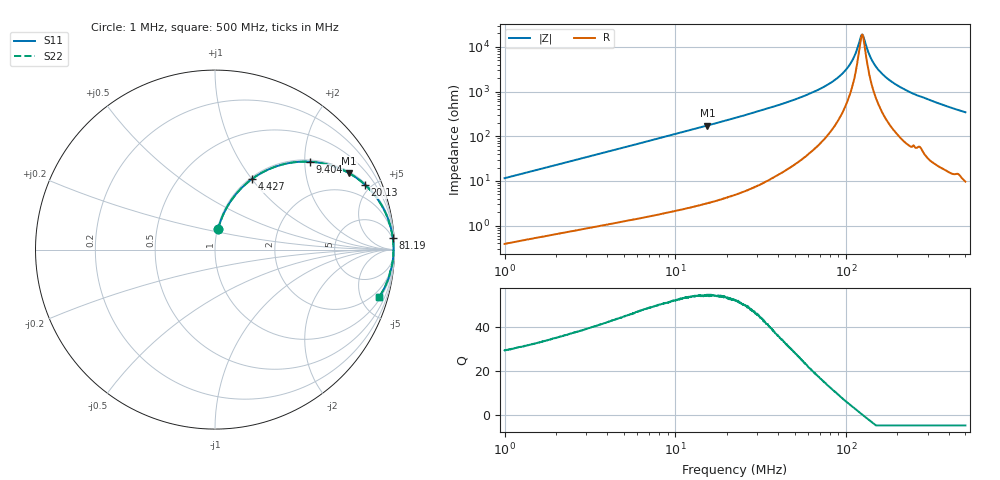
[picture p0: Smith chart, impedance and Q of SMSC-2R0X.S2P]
!s-Parameter Generated by FASTRON Sdn. Bhd.
!FASTRON P/N : SMSC-2R0X
!Keysight Technologies,E4991B,MY54100416,A.01.15
!Date: Mon Mar 16 10:09:13 2026
!Version  : Rev00 Mon Mar 16 10:09:13 2026
!Data & Calibration Information:
!PortZ  Port1:50+j0  Port2:50+j0
!When reading, reference impedance value at option line is always used.
! Remarks : This data is being provided solely for informational purposes.
!Freq	S11	S21	S12	S22
# Hz S dB R 50
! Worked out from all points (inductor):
!   1601 points, 1 MHz to 500 MHz, reference 50 ohm
!   read as one part in series: L = 1.83 uH near 1.032 MHz
!   highest Q = 54.8 at 15.4 MHz (marker M1), where L = 1.8 uH
!   self-resonance near 124 MHz
!   S11 on the Smith chart (normalised r, x): 1 MHz: 1.01, +0.23; 4.427 MHz: 1.02, +1.00; 9.404 MHz: 1.04, +2.11; 20.13 MHz: 1.09, +4.59; 81.19 MHz: 4, +31; 500 MHz: 1.19, -6.89
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1000000  -18.84 81.5  -0.09 -6.6  -0.09 -6.6  -18.84 81.5
2820919  -10.39 70.9  -0.49 -17.6  -0.49 -17.6  -10.39 70.9
4426556  -7.08 62.4  -1.04 -26.3  -1.04 -26.3  -7.08 62.4
7957584  -3.61 47.6  -2.63 -41.3  -2.63 -41.3  -3.61 47.6
9404074  -2.86 42.9  -3.34 -46.0  -3.34 -46.0  -2.86 42.9
1.540092e7  -1.31 29.6  -6.12 -59.3  -6.12 -59.3  -1.31 29.6
2.013446e7  -0.81 23.3  -8.04 -65.6  -8.04 -65.6  -0.81 23.3
2.236068e7  -0.67 21.1  -8.86 -67.8  -8.86 -67.8  -0.67 21.1
4.05111e7  -0.21 11.2  -14.25 -77.2  -14.25 -77.2  -0.21 11.2
6.307767e7  -0.09 6.0  -19.57 -81.2  -19.57 -81.2  -0.09 6.0
8.11935e7  -0.06 3.6  -23.96 -81.7  -23.96 -81.7  -0.06 3.6
9.374216e7  -0.05 2.4  -27.64 -80.4  -27.64 -80.4  -0.05 2.4
1.045122e8  -0.05 1.4  -31.78 -76.7  -31.78 -76.7  -0.05 1.4
1.116461e8  -0.05 0.9  -35.65 -70.6  -35.65 -70.6  -0.05 0.9
1.211344e8  -0.05 0.2  -43.78 -35.1  -43.78 -35.1  -0.05 0.2
1.239906e8  -0.05 0.0  -45.45 -3.7  -45.45 -3.7  -0.05 0.0
1.269141e8  -0.05 -0.2  -44.30 29.4  -44.30 29.4  -0.05 -0.2
1.366344e8  -0.05 -0.8  -36.65 68.0  -36.65 68.0  -0.05 -0.8
1.459609e8  -0.05 -1.3  -32.40 75.6  -32.40 75.6  -0.05 -1.3
1.77937e8  -0.06 -3.1  -25.42 81.0  -25.42 81.0  -0.06 -3.1
2.51418e8  -0.12 -6.4  -18.99 79.7  -18.99 79.7  -0.12 -6.4
5e8  -0.42 -16.0  -11.17 72.3  -11.17 72.3  -0.42 -16.0
